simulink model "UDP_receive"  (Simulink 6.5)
settings: Solver=FixedStepDiscrete  SolverMode=SingleTasking  StartTime=0.0  StopTime=inf  FixedStep=.002  RelTol=1e-3
libraries: xpclib x2

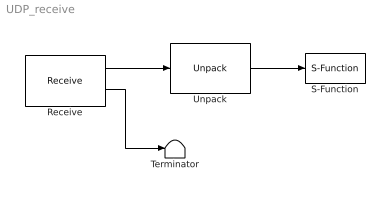
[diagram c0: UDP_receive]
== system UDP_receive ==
  Receive : xpclib/UDP/Receive  ipAddress=132.206.111.69  ipPort=5000  width=8*5  sampletime=0.02
  S-Function : S-Function  FunctionName=UDP_plot
  Terminator : Terminator
  Unpack : xpclib/UDP/Unpack  dimensions={[5]}  datatypes={'double'}  byteAlign=1
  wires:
  Receive/1 -> Unpack/1
  Unpack/1 -> S-Function/1
  Receive/2 -> Terminator/1
